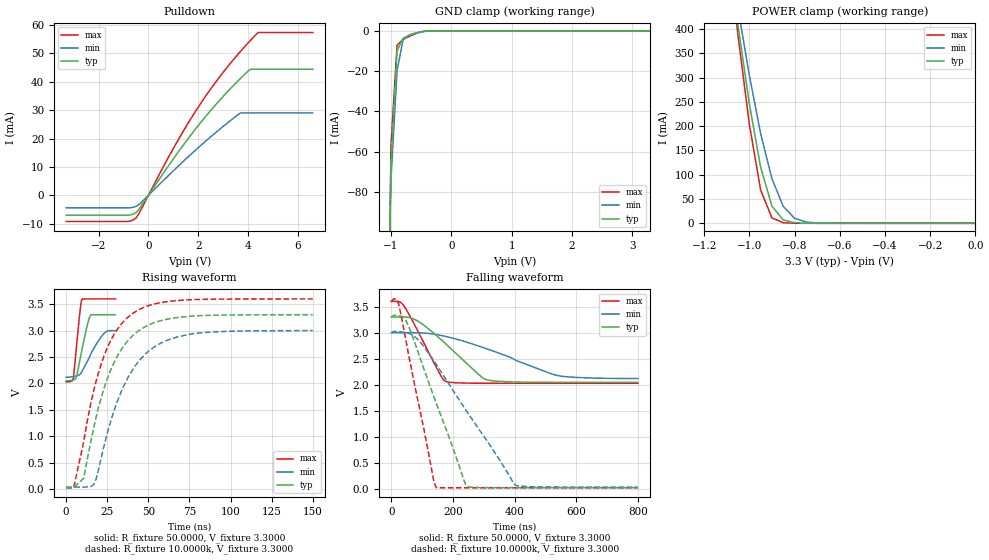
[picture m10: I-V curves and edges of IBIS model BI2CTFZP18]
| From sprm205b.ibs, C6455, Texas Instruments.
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|   Model BI2CTFZP18
[Model]   BI2CTFZP18
Model_type   I/O_open_drain
Polarity   Non-Inverting
Enable   Active-Low
Vinl =   0.8000V
Vinh =   2.0000V
Vmeas =  1.6500V
Cref =   5.0000pF
Rref =   10k
Vref =   3.3000V
C_comp   1.3060pF   1.2089pF   1.4160pF
[Temperature Range]   25.0000   0.1250k   -40.0000
[Voltage Range]   3.3000V   3.0000V   3.6000V
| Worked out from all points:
|   slope of the pulldown table from 0 to 0.495 V, typ, clamps not added: 76.9 ohm
|   GND clamp passes 1 mA (typ) near -0.57 V on its own axis
|   POWER clamp passes 1 mA (typ) near -0.79 V on its own axis
|   rising waveform, R_fixture 50.0000, V_fixture 3.3000: 20-80 % time 4.99ns typ, 9.22ns min, 2.95ns max; typ from 2.05 V to 3.3 V
|   rising waveform, R_fixture 10.0000k, V_fixture 3.3000: 20-80 % time 20ns typ, 22.2ns min, 18.8ns max; typ from 0.025 V to 3.3 V
|   falling waveform, R_fixture 50.0000, V_fixture 3.3000: 20-80 % time 139ns typ, 240ns min, 82ns max; typ from 3.3 V to 2.05 V
|   falling waveform, R_fixture 10.0000k, V_fixture 3.3000: 20-80 % time 120ns typ, 200ns min, 72.7ns max; typ from 3.3 V to 0.025 V
[Pulldown]
| voltage   I(typ)   I(min)   I(max)
-3.3V     -6.968mA   -4.387mA   -9.211mA
-800mV    -6.968mA   -4.387mA   -9.155mA
-600mV    -6.559mA   -4.141mA   -8.631mA
-500mV    -6.09mA    -3.872mA   -7.986mA
-300mV    -3.926mA   -2.619mA   -5.079mA
1V        12.83mA    8.625mA    16.48mA
1.5V      18.86mA    12.78mA    24.05mA
1.9V      23.44mA    15.99mA    29.68mA
2.8V      32.89mA    22.83mA    41.01mA
3.7V      41.2mA     29.01mA    50.7mA
4.1V      44.39mA    NA         54.57mA
6.6V      44.39mA    29.01mA    57.3mA
[GND_clamp]
| voltage   I(typ)   I(min)   I(max)
-3.3V     -13.47A    -11.36A    -15.18A
-1.1V     -233.8mA   -193.9mA   -288.4mA
-1V       -63.72mA   -73.58mA   -56.37mA
-900mV    -9.894mA   -19.89mA   -7.141mA
-800mV    -3.664mA   -4.378mA   -4.275mA
-700mV    -2.327mA   -2.082mA   -2.798mA
-500mV    -447.7uA   -521.6uA   -455.2uA
-400mV    -55.53uA   -127.7uA   -42.22uA
3.3V      40.72nA    62.96nA    139nA
[POWER_clamp]
| voltage   I(typ)   I(min)   I(max)
-3.3V     9.936A     8.46A      11.24A
-1.1V     585mA      590.8mA    591.8mA
-1.05V    407.3mA    442.4mA    386.8mA
-1V       246.3mA    305mA      204.2mA
-950mV    115.4mA    184.9mA    68.68mA
-900mV    35.32mA    91.75mA    11.02mA
-850mV    7.005mA    34.84mA    1.147mA
-800mV    1.172mA    10.42mA    109.9uA
-750mV    189.3uA    2.784mA    10.24uA
-650mV    4.599uA    191.8uA    288.9nA
0V        40.72nA    31.33nA    149nA
[Ramp]
| variable   typ   min   max
dV/dt_r   5.4252u/22.9109n  1.5618u/31.8807n  18.0726u/15.8908n
dV/dt_f   0.7524/0.1379u   0.5292/0.2459u   0.9433/81.1224n
R_load = 50.0000
[Rising Waveform]
R_fixture = 50.0000
V_fixture = 3.3000
V_fixture_min = 3.0000
V_fixture_max = 3.6000
| time   V(typ)   V(min)   V(max)
0s        2.046V     2.115V     2.028V
4.242ns   2.063V     2.128V     2.077V
6.364ns   2.135V     2.141V     2.723V
8.485ns   2.46V      2.174V     3.384V
9.091ns   2.554V     2.197V     3.53V
9.697ns   2.648V     2.229V     3.594V
13.03ns   3.125V     2.428V     3.6V
14.85ns   3.289V     2.542V     3.6V
23.03ns   3.3V       2.944V     3.6V
30ns      3.3V       2.999V     3.6V
[Rising Waveform]
R_fixture = 10.0000k
V_fixture = 3.3000
V_fixture_min = 3.0000
V_fixture_max = 3.6000
| time   V(typ)   V(min)   V(max)
0s        25.02mV    33.88mV    21.16mV
4.546ns   24.8mV     33.81mV    20.7mV
10.61ns   199.5mV    35.64mV    882.2mV
16.67ns   1.146V     79.09mV    1.847V
21.21ns   1.717V     575.9mV    2.357V
27.27ns   2.267V     1.301V     2.821V
39.39ns   2.87V      2.207V     3.3V
51.52ns   3.124V     2.643V     3.486V
69.7ns    3.254V     2.893V     3.572V
150ns     3.3V       2.999V     3.599V
[Falling Waveform]
R_fixture = 50.0000
V_fixture = 3.3000
V_fixture_min = 3.0000
V_fixture_max = 3.6000
| time   V(typ)   V(min)   V(max)
0s        3.3V       3V         3.6V
24.24ns   3.3V       3V         3.597V
40.4ns    3.299V     3V         3.518V
88.89ns   3.21V      2.997V     2.996V
161.6ns   2.864V     2.946V     2.164V
177.8ns   2.777V     2.925V     2.061V
282.8ns   2.2V       2.744V     2.029V
315.2ns   2.086V     2.678V     2.028V
541.4ns   2.046V     2.174V     2.028V
800ns     2.046V     2.118V     2.028V
[Falling Waveform]
R_fixture = 10.0000k
V_fixture = 3.3000
V_fixture_min = 3.0000
V_fixture_max = 3.6000
| time   V(typ)   V(min)   V(max)
0s        3.3V       3V         3.599V
16.16ns   3.331V     3.02V      3.642V
24.24ns   3.328V     3.017V     3.544V
56.57ns   3.117V     2.987V     2.567V
88.89ns   2.591V     2.85V      1.623V
137.4ns   1.777V     2.464V     163mV
145.5ns   1.648V     2.392V     26.11mV
242.4ns   66.92mV    1.509V     21.29mV
404ns     25.32mV    67.96mV    21.16mV
800ns     25.02mV    34.09mV    21.16mV
